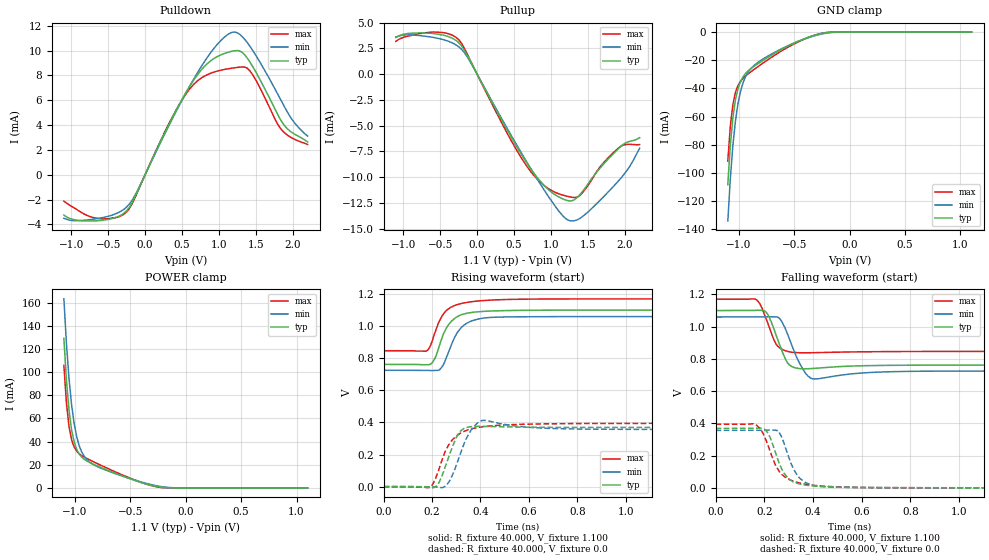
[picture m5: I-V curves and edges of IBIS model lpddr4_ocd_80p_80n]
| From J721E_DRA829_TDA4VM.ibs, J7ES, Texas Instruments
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|   Model lpddr4_ocd_80p_80n
[Model] lpddr4_ocd_80p_80n
Model_type I/O
Polarity   Non-Inverting
Enable   Active-High
Vinl =  0.113V
Vinh =  0.253V
Vmeas =  0.183V
C_comp   2.243pF   2.045pF   2.499pF
[Model Spec]
Vinh   0.253V   0.247V   0.265V
Vinl   0.113V   0.107V   0.125V
Vmeas   0.183V   0.176V   0.195V
[Temperature Range]   25.000   0.125k   -40.000
[Voltage Range]   1.100V   1.060V   1.170V
[Pullup Reference]   1.100V   1.060V   1.170V
[Pulldown Reference]   0.0V   0.0V   0.0V
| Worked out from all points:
|   slope of the pulldown table from 0 to 0.165 V, typ, clamps not added: 77.8 ohm
|   slope of the pullup table from 0 to 0.165 V, typ, clamps not added: 73.7 ohm
|   GND clamp passes 1 mA (typ) near -0.25 V on its own axis
|   POWER clamp passes 1 mA (typ) near -0.26 V on its own axis
|   rising waveform, R_fixture 40.000, V_fixture 1.100: 20-80 % time 61ps typ, 65.6ps min, 63.9ps max; typ from 0.762 V to 1.1 V
|   rising waveform, R_fixture 40.000, V_fixture 0.0: 20-80 % time 54ps typ, 53.4ps min, 79.1ps max; typ from 0 V to 0.369 V
|   falling waveform, R_fixture 40.000, V_fixture 1.100: 20-80 % time 50.1ps typ, 54ps min, 48.3ps max; typ from 1.1 V to 0.762 V
|   falling waveform, R_fixture 40.000, V_fixture 0.0: 20-80 % time 61.3ps typ, 60.6ps min, 74.1ps max; typ from 0.369 V to 0 V
[Pulldown]
|Voltage   I(typ)   I(min)   I(max)
-1.1V     -3.255mA   -3.506mA   -2.125mA
-692mV    -3.717mA   -3.57mA    -3.462mA
-284mV    -3.081mA   -2.767mA   -3.161mA
-113mV    -1.48mA    -1.385mA   -1.522mA
295mV     3.732mA    3.634mA    3.789mA
567mV     6.767mA    6.746mA    6.623mA
839mV     8.929mA    9.426mA    8.05mA
1.179V    9.946mA    11.47mA    8.583mA
1.384V    9.383mA    10.63mA    8.573mA
1.826V    4.503mA    6.14mA     3.777mA
1.996V    3.366mA    4.383mA    2.934mA
2.2V      2.638mA    3.112mA    2.436mA
[Pullup]
|Voltage   I(typ)   I(min)   I(max)
-1.1V     3.559mA    3.612mA    3.186mA
-590mV    3.943mA    3.564mA    4.09mA
-249mV    3.061mA    2.656mA    3.35mA
-113mV    1.558mA    1.447mA    1.658mA
397mV     -5.297mA   -5.132mA   -5.598mA
669mV     -8.585mA   -8.493mA   -8.902mA
975mV     -11.27mA   -11.98mA   -11.17mA
1.247V    -12.32mA   -14.22mA   -11.91mA
1.384V    -11.77mA   -14.05mA   -11.84mA
1.69V     -8.911mA   -12.07mA   -8.796mA
1.928V    -7.122mA   -10.26mA   -7.105mA
2.2V      -6.17mA    -7.201mA   -6.842mA
[GND_clamp]
|Voltage   I(typ)   I(min)   I(max)
-1.1V     -108.4mA   -134.2mA   -91.64mA
-1.077V   -80.17mA   -103.9mA   -66.63mA
-1.054V   -60.68mA   -80.47mA   -51.43mA
-1.031V   -48.01mA   -63.16mA   -42.83mA
-1.008V   -40.05mA   -50.75mA   -37.96mA
-985mV    -35.04mA   -42.04mA   -34.98mA
-940mV    -29.42mA   -31.64mA   -31.22mA
-894mV    -26.11mA   -26.16mA   -28.35mA
-848mV    -23.5mA    -22.73mA   -25.7mA
-527mV    -8.739mA   -8.686mA   -9.514mA
-229mV    -630.6uA   -1.042mA   -565.6uA
1.1V      0A         0A         0A
[POWER_clamp]
|Voltage   I(typ)   I(min)   I(max)
-1.1V     129.2mA    163.4mA    105.9mA
-1.077V   92.86mA    124.8mA    73.4mA
-1.054V   67.3mA     94.73mA    53.17mA
-1.031V   50.48mA    72.25mA    41.67mA
-1.008V   39.92mA    56.03mA    35.37mA
-985mV    33.38mA    44.6mA     31.76mA
-963mV    29.31mA    36.69mA    29.53mA
-917mV    24.75mA    27.38mA    26.61mA
-871mV    22.09mA    22.57mA    24.31mA
-619mV    11.98mA    11.76mA    13.12mA
-229mV    602.6uA    1.183mA    400.7uA
1.1V      0A         0A         0A
[Ramp]
| variable   typ   min   max
dV/dt_r   0.221/53.888p   0.214/52.921p   0.237/78.981p
dV/dt_f   0.204/50.282p   0.201/53.670p   0.194/48.116p
R_load = 40.000
[Rising Waveform]
R_fixture= 40.000
V_fixture= 1.100
V_fixture_min= 1.060
V_fixture_max= 1.170
|time   V(typ)   V(min)   V(max)
0s        761.9mV    725.2mV    847mV
177ps     760mV      725.1mV    845.7mV
193ps     762.9mV    723.5mV    876.5mV
205ps     780.8mV    723.7mV    929.3mV
226ps     857.8mV    724.9mV    1.018V
252ps     968.3mV    775.6mV    1.085V
286ps     1.04V      906.2mV    1.124V
331ps     1.076V     1.005V     1.144V
400ps     1.091V     1.047V     1.158V
3ns       1.1V       1.06V      1.17V
[Rising Waveform]
R_fixture= 40.000
V_fixture= 0.0
V_fixture_min= 0.0
V_fixture_max= 0.0
|time   V(typ)   V(min)   V(max)
0s        389.4uV    699uV      674uV
191ps     -4.455mV   -832.7uV   -3.175mV
223ps     12.21mV    -2.03mV    84.31mV
253ps     115.7mV    437.1uV    215.3mV
282ps     239.4mV    64.13mV    287.5mV
315ps     342.8mV    198.7mV    331.7mV
359ps     374.2mV    347.8mV    358.8mV
415ps     375.7mV    414mV      374.8mV
788ps     369.2mV    359.6mV    393.3mV
3ns       369mV      356.9mV    395mV
[Falling Waveform]
R_fixture= 40.000
V_fixture= 1.100
V_fixture_min= 1.060
V_fixture_max= 1.170
|time   V(typ)   V(min)   V(max)
0s        1.1V       1.06V      1.17V
166ps     1.102V     1.06V      1.169V
210ps     1.086V     1.061V     1.04V
238ps     992.7mV    1.061V     922.8mV
258ps     909.4mV    1.057V     875.4mV
302ps     764mV      929.8mV    844.6mV
354ps     738.7mV    747.5mV    837.7mV
406ps     741.5mV    675.1mV    838.6mV
793ps     760.8mV    722.7mV    845.9mV
3ns       761.9mV    725.2mV    847mV
[Falling Waveform]
R_fixture= 40.000
V_fixture= 0.0
V_fixture_min= 0.0
V_fixture_max= 0.0
|time   V(typ)   V(min)   V(max)
0s        369mV      356.9mV    395mV
168ps     370.8mV    356.8mV    389.2mV
195ps     368.5mV    357.3mV    339.1mV
215ps     340mV      358.4mV    263.6mV
253ps     188.2mV    355.7mV    122.4mV
269ps     127.2mV    323.7mV    90.27mV
289ps     75.67mV    241.2mV    64.01mV
335ps     28.91mV    79.55mV    34.22mV
422ps     9.447mV    10.54mV    13.25mV
3ns       389.3uV    698uV      674uV
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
